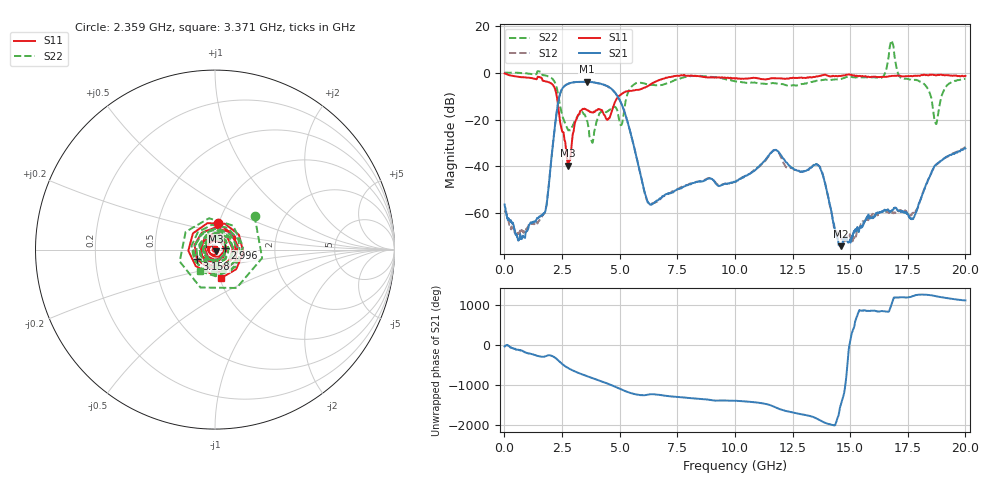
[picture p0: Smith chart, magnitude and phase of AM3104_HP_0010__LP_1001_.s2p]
!Created with skrf (http://scikit-rf.org).
# Hz S RI R 50.0
!freq ReS11 ImS11 ReS21 ImS21 ReS12 ImS12 ReS22 ImS22
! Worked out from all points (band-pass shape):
!   1601 points, 10 MHz to 20 GHz, reference 50 ohm
!   highest |S21| = -3.91 dB at 3.571 GHz (marker M1); lowest = -73.9 dB at 14.59 GHz (marker M2)
!   |S21| within 3 dB of the highest: 2.508 GHz to 4.644 GHz (2.136 GHz wide, 59.7 % of centre)
!   lowest |S11| = -39.7 dB at 2.771 GHz (marker M3), VSWR 1.02, Z = 50.4 - j0.971 ohm
!   |S11| at or under -10 dB: 2.272 GHz to 4.974 GHz (2.702 GHz wide, 74.6 % of centre)
!   |S22| runs from -29.9 to 13.7 dB; largest |S21 - S12| = 0.048
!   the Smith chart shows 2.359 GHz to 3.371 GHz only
!   S11 on the Smith chart (normalised r, x): 2.359 GHz: 0.99, +0.30; 2.996 GHz: 1.11, +0.02; 3.158 GHz: 0.81, -0.09; 3.371 GHz: 1.01, -0.33
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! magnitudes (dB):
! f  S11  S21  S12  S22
! 10 MHz  -0.4  -56.2  -58.8  0.0
! 672.2 MHz  -1.9  -70.1  -68.5  -0.2
! 1.722 GHz  -3.6  -60.0  -60.1  -1.2
! 2.359 GHz  -16.5  -11.4  -11.5  -10.7
! 2.771 GHz  -39.7  -4.8  -4.8  -24.6
! 2.996 GHz  -25.3  -4.2  -4.2  -22.0
! 3.158 GHz  -18.9  -4.0  -4.0  -19.1
! 3.346 GHz  -16.0  -4.0  -4.0  -16.7
! 3.371 GHz  -15.8  -4.0  -4.0  -16.6
! 3.571 GHz  -15.9  -3.9  -4.0  -20.4
! 4.908 GHz  -10.7  -10.1  -10.1  -16.5
! 6.169 GHz  -6.1  -53.6  -54.0  -4.9
! 6.682 GHz  -3.3  -54.2  -54.4  -5.5
! 10.01 GHz  -2.5  -46.7  -46.6  -3.7
! 11.72 GHz  -2.5  -33.1  -33.1  -4.5
! 13.34 GHz  -2.1  -40.2  -40.1  -4.0
! 13.77 GHz  -1.2  -42.2  -41.9  -3.2
! 14.59 GHz  -1.5  -73.9  -69.5  -2.8
! 16.68 GHz  -1.6  -58.9  -59.7  7.3
! 17.74 GHz  -1.4  -62.3  -59.6  -3.1
! 18.71 GHz  -1.2  -39.3  -39.4  -21.7
! 20 GHz  -1.4  -32.3  -31.8  -2.6
